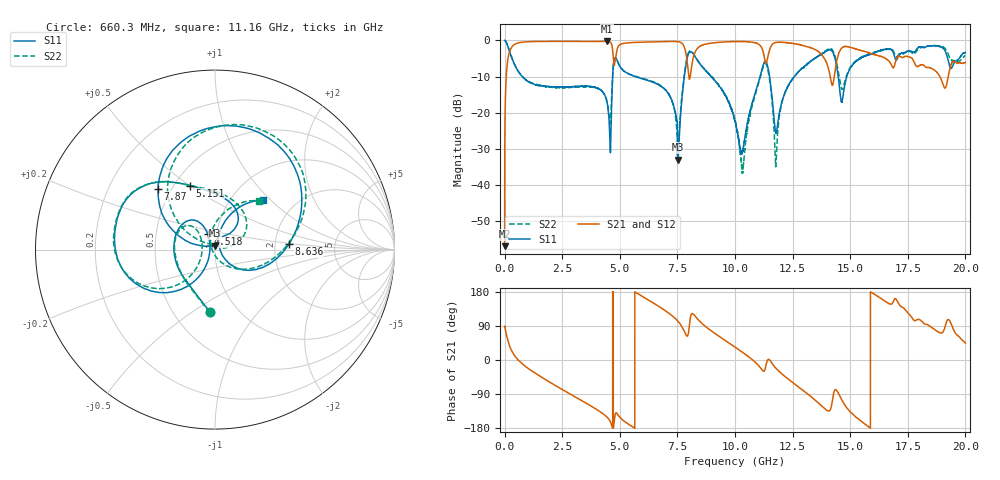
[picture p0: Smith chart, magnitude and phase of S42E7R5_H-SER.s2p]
!{S42E7R5}
!Johanson Technology Inc.
!www.johansontechnology.com
!Test Board Conditions:
!Substrate Type  RO4350B
!Substrate Thickness  50 mil
!Substrate Dk  3.66
!TL Type: GCPW
!TL Trace Width  60 mil
!TL Gap  10 mil
!Electrode orientation  Horizontal
!DUT TOPOLOGY	SERIES
!Mounting Pad LxW  14x55 mil
! Created Wed Nov 25 21:50:34 2020
# khz S ma R 50
! 2 Port Network Data from SP1.SP block
! freq  magS11  angS11  magS21  angS21  magS12  angS12  magS22  angS22
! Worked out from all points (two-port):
!   20001 points, 300 kHz to 20 GHz, reference 50 ohm
!   highest |S21| = -0.24 dB at 4.435 GHz (marker M1); lowest = -56.9 dB at 300 kHz (marker M2)
!   |S21| within 3 dB of the highest: 208.8 MHz to 4.698 GHz (4.489 GHz wide, 183 % of centre); 4.853 GHz to 7.862 GHz (3.008 GHz wide, 47.3 % of centre)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
!   lowest |S11| = -32.9 dB at 7.521 GHz (marker M3), VSWR 1.05, Z = 49.7 + j2.23 ohm
!   |S11| at or under -10 dB: 770.5 MHz to 4.69 GHz (3.92 GHz wide, 144 % of centre); 5.676 GHz to 7.798 GHz (2.122 GHz wide, 31.5 % of centre); 8.968 GHz to 11.09 GHz (2.12 GHz wide, 21.1 % of centre)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
!   |S22| runs from -36.9 to 0.0 dB; largest |S21 - S12| = 0.016
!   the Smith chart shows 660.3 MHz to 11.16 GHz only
!   S11 on the Smith chart (normalised r, x): 660.3 MHz: 0.75, -0.59; 4.518 GHz: 0.91, +0.16; 5.151 GHz: 0.60, +0.50; 7.87 GHz: 0.43, +0.37; 8.636 GHz: 2.39, +0.17; 11.16 GHz: 1.39, +0.90
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300  0.9998 -0.3  0.001434 87.7  0.001314 90.3  0.9966 -0.0
146300  0.8245 -39.5  0.5589 50.3  0.5608 50.1  0.8259 -39.5
660300  0.3483 -94.3  0.9344 -4.2  0.9351 -4.1  0.3501 -94.7
3334300  0.2326 158.7  0.9693 -106.9  0.9683 -106.8  0.2285 167.2
4435300  0.145 116.3  0.973 -150.1  0.972 -150.1  0.1491 133.0
4518300  0.09419 115.0  0.9666 -155.8  0.9668 -155.8  0.106 139.3
4791300  0.5677 168.0  0.5151 -145.3  0.516 -145.5  0.5732 166.6
5151300  0.384 111.6  0.9098 -159.6  0.91 -159.7  0.3849 111.5
6667300  0.2451 60.4  0.9597 142.3  0.958 142.3  0.2487 47.1
7521300  0.02258 96.0  0.9631 102.6  0.9629 102.7  0.02699 101.1
7870300  0.4629 133.2  0.6666 66.4  0.6647 66.3  0.4857 121.8
8636300  0.4123 4.1  0.8734 92.7  0.8725 92.7  0.4147 5.3
1.00003e7  0.07672 -43.7  0.965 34.0  0.9674 34.0  0.08035 -63.7
1.03383e7  0.02976 37.2  0.9646 19.8  0.9645 19.8  0.01639 -179.3
1.11603e7  0.3846 45.9  0.7903 -24.9  0.7867 -24.8  0.3658 48.2
1.14473e7  0.3982 -30.9  0.6378 1.7  0.6388 2.0  0.3664 -38.4
1.17853e7  0.05265 0.5  0.9396 -22.2  0.939 -22.3  0.02143 16.0
1.33343e7  0.5271 -3.5  0.782 -98.3  0.7878 -98.2  0.5301 -15.7
1.41803e7  0.7352 -72.9  0.2634 -123.1  0.2661 -123.3  0.7615 -78.1
1.46403e7  0.1403 -70.2  0.7899 -105.7  0.7916 -105.5  0.2123 -85.1
1.66673e7  0.7606 -120.2  0.5247 149.5  0.512 149.8  0.7626 -129.8
2e7  0.6809 148.6  0.4974 44.4  0.4991 45.2  0.6165 131.2
